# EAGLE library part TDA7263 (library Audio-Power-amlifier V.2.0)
The TDA7263 is class AB dual audio power amplifier assembled in the new Clipwatt package, specially designed for high quality sound application as HI-FI music centers and stereo TV sets.
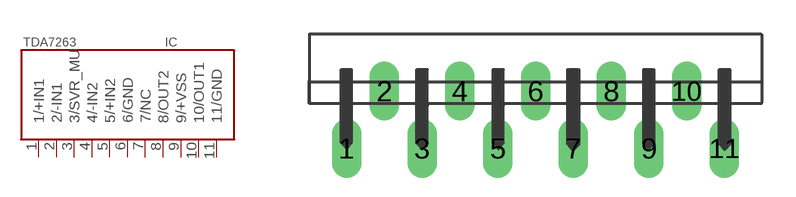
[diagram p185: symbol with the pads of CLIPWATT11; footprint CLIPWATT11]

Designator prefix IC

## TDA7263  [CLIPWATT11]
1  1/+IN1  in
2  2/-IN1  in
3  3/SVR_MU  in
4  4/-IN2  in
5  5/+IN2  in
6  6/GND  pwr
7  7/NC  nc
8  8/OUT2  out
9  9/+VSS  pwr
10  10/OUT1  out
11  11/GND  nc

## Footprint CLIPWATT11 (pad centres in mm)
drill 0.8 long: 1 -8.382,0; 2 -6.706,2.54; 3 -5.029,0; 4 -3.353,2.54; 5 -1.676,0; 6 0,2.54; 7 1.676,0; 8 3.353,2.54; 9 5.029,0; 10 6.706,2.54; 11 8.382,0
